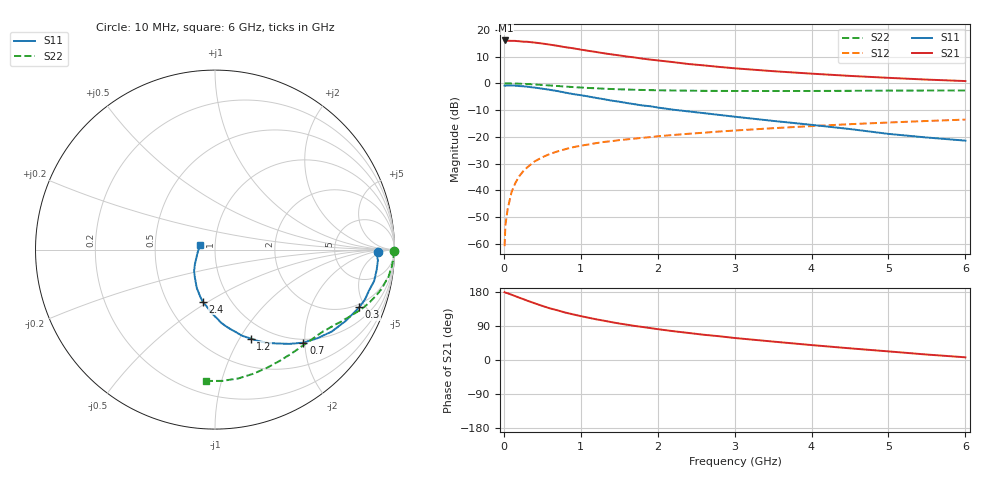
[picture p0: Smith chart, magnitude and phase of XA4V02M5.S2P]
! SIEMENS Discrete & RF Semiconductors
! BFY180
! Si NPN RF Bipolar Junction Transistor in MICRO-X
! VCE = 4 V  IC = 2.5 mA
! Common Emitter S-Parameters:  May  1997
# GHz  S  MA  R  50
!  f  S11  S21  S12  S22
! GHz  MAG  ANG  MAG  ANG  MAG  ANG  MAG  ANG
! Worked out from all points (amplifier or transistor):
!   36 points, 10 MHz to 6 GHz, reference 50 ohm
!   highest |S21| = 16.0 dB at 20 MHz (marker M1)
!   |S21| within 3 dB of that: start of sweep to 915.9 MHz
!   unconditionally stable (mu >= 1): 2.572 GHz to end of sweep
!   at 250 MHz: K = 0.13, MSG = 24.3 dB, |S12| = -33.0 dB
!   at 1.4 GHz: K = 0.73, MSG = 16.2 dB, |S12| = -21.6 dB
!   at 6 GHz: K = 1.06, MAG = 5.7 dB, |S12| = -13.6 dB
!   S11 on the Smith chart (normalised r, x): 10 MHz: 21, -3; 300 MHz: 1.77, -4.53; 700 MHz: 0.93, -1.97; 1.2 GHz: 0.81, -1.12; 2.4 GHz: 0.74, -0.47; 6 GHz: 0.85, +0.04
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0.01  0.9093 -0.7  6.233 178.8  0.0009 92.7  0.9953 -0.3
0.02  0.901 -1.6  6.331 177.9  0.0022 94.4  0.9957 -0.7
0.05  0.9098 -3.7  6.245 176.1  0.0045 85.2  0.9959 -1.8
0.1  0.9077 -7.3  6.223 172.3  0.0092 85.8  0.993 -3.6
0.15  0.9033 -11.3  6.209 168.4  0.0137 83.4  0.9898 -5.4
0.3  0.8657 -21.8  5.985 156.9  0.0265 76.9  0.9687 -10.4
0.5  0.7946 -35.1  5.546 142.8  0.0414 69.3  0.9307 -16.3
0.6  0.7545 -40.9  5.285 136.2  0.0479 65.8  0.9105 -18.8
0.7  0.7149 -46.5  5.021 131.0  0.0534 62.9  0.8899 -21.1
0.8  0.6693 -51.7  4.737 125.1  0.0587 60.8  0.8696 -23.2
0.9  0.6296 -56.2  4.523 120.4  0.0638 57.9  0.8506 -25.1
1.1  0.567 -64.3  4.048 111.6  0.0718 54.8  0.8189 -28.4
1.2  0.5335 -68.2  3.851 107.4  0.0761 53.1  0.8064 -30.1
1.5  0.4526 -78.8  3.326 96.3  0.0865 49.6  0.7731 -34.3
1.7  0.4068 -85.5  3.044 90.0  0.0924 48.1  0.7558 -37.0
2.2  0.3214 -98.1  2.491 76.1  0.108 44.3  0.734 -43.4
2.4  0.2982 -103.3  2.296 71.4  0.1138 42.9  0.7279 -46.0
3  0.2375 -115.2  1.91 58.1  0.1308 39.1  0.719 -53.4
3.5  0.1982 -124.0  1.686 48.6  0.1448 36.1  0.7172 -59.6
4.5  0.1395 -143.5  1.376 30.8  0.1721 28.8  0.7237 -72.8
5.5  0.0969 -172.3  1.173 14.4  0.1975 21.2  0.7325 -86.8
6  0.0847 162.7  1.102 7.1  0.2097 16.9  0.7335 -93.8
